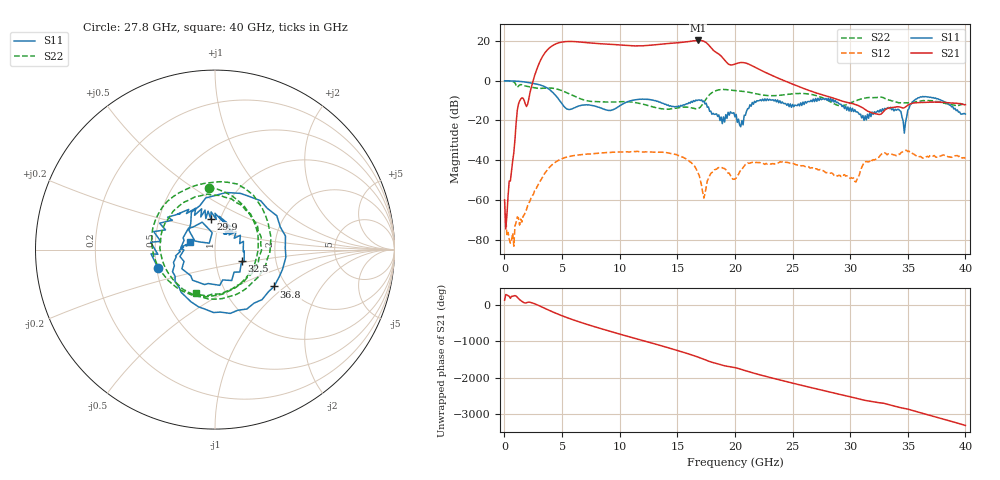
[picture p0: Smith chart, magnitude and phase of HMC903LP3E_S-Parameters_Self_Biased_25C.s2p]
! Hittite Microwave Corporation
! 20 Alpha Road
! Chelmsford, MA 01824
! http://www.hittite.com
! Tel: 978-250-3343
! Fax: 978-250-3373
! Device:  HMC903LP3E
! Description: GaAs pHEMT MMIC Low Noise Amplifier
! Frequency:  6.00 -  17.00 GHz
! Package:  LP3  - 3x3 mm Quad Flatpack No-Lead (QFN) Plastic Package: 16 pin
! Ports:  2 RF, 4 DC
!  Pin  3 = RF In  = Port 1
!  Pin  5 = Vgg1 (Optional)
!  Pin  6 = Vgg2 (Optional)
!  Pin 10 = RF Out  = Port 2
!  Pin 14 = Vdd2
!  Pin 15 = Vdd1
! Voltages:  Vdd  = Vdd1 = Vdd2 = +3.50  Volts
!  Idd  = Idd1 + Idd2 = 87.08  mA
!  Vgg1  = left opened
!  Vgg2  = left opened
! Data:  The device was measured on evaluation board 128395.
! Board loss de-embedded from S21 magnitude. All other RF measurements reference to RF coaxial connector.
! Misc:
! Date Measured:  2010-2-16
! Date:
! Note:
!  Hittite supplies this data as a sample of measured data at the package pin for
!  for this package product.  Your particular data for this product may vary.
!  Data was taken at 25 degrees C.
!  Hittite reserves the right to change this data at anytime.
# GHz S DB R 50
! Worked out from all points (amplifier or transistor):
!   401 points, 10 MHz to 40 GHz, reference 50 ohm
!   highest |S21| = 20.1 dB at 16.81 GHz (marker M1)
!   |S21| within 3 dB of that: 4.065 GHz to 17.83 GHz (13.77 GHz wide, 126 % of centre)
!   unconditionally stable (mu >= 1): start of sweep to end of sweep
!   at 6.608 GHz: K = 3.35, MAG = 20.1 dB, |S12| = -37.2 dB
!   at 20 GHz: K = 38.41, MAG = 10.0 dB, |S12| = -49.4 dB
!   at 40 GHz: K = 164.99, MAG = -11.7 dB, |S12| = -39.1 dB
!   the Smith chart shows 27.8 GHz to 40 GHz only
!   S11 on the Smith chart (normalised r, x): 27.8 GHz: 0.51, -0.12; 29.9 GHz: 0.90, +0.32; 32.5 GHz: 1.33, -0.18; 36.8 GHz: 1.73, -0.83; 40 GHz: 0.76, +0.07
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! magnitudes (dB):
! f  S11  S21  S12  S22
! 10 MHz  -0.1  -59.9  -67.1  -0.1
! 309.9 MHz  -0.1  -58.0  -76.2  -0.2
! 609.9 MHz  -0.2  -45.2  -80.2  -0.3
! 1.31 GHz  -0.4  -10.3  -72.5  -2.2
! 2.01 GHz  -0.9  -11.9  -62.8  -2.9
! 3.809 GHz  -4.1  15.9  -44.2  -3.7
! 6.708 GHz  -12.4  19.3  -37.2  -9.4
! 13.41 GHz  -10.8  18.2  -36.0  -13.9
! 16.81 GHz  -9.7  20.1  -46.4  -14.0
! 17.31 GHz  -10.2  19.7  -59.0  -10.9
! 18.51 GHz  -18.0  13.7  -43.9  -4.8
! 20.1 GHz  -17.0  8.5  -49.0  -5.1
! 21.5 GHz  -11.0  7.4  -41.1  -6.2
! 26.7 GHz  -10.6  -5.5  -43.7  -7.0
! 27.8 GHz  -9.5  -7.5  -45.8  -9.2
! 29.9 GHz  -15.3  -11.2  -48.3  -11.5
! 32.5 GHz  -15.8  -17.0  -38.5  -8.4
! 33.4 GHz  -14.0  -13.7  -36.8  -9.8
! 34.7 GHz  -26.4  -13.6  -35.2  -11.2
! 35.4 GHz  -10.7  -11.4  -36.6  -10.9
! 36.8 GHz  -8.2  -10.9  -38.5  -10.0
! 40 GHz  -16.8  -12.1  -39.1  -11.5
